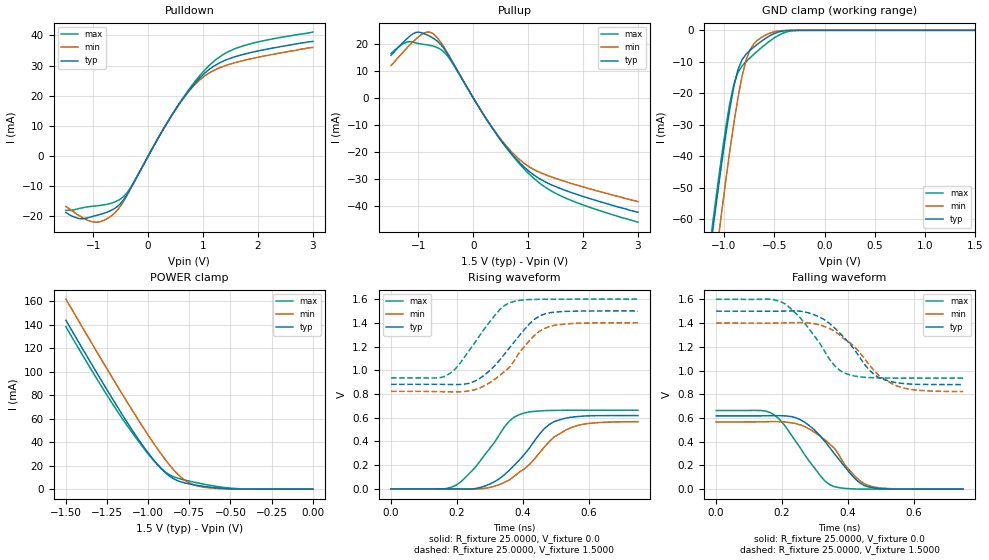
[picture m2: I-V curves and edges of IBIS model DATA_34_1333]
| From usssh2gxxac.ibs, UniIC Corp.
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|   Model DATA_34_1333
[Model]  DATA_34_1333
Model_type I/O
Polarity   Non-Inverting
Enable   Active-High
Vinl =   0.60000000V
Vinh =   0.90000000V
Vmeas =   0.750000000V
Rref =   25.00000000
Vref =   0.75000000V
C_comp   1.6160pF   1.5990pF   1.6430pF
[Temperature Range]   25.0000   95.0000   0.0
[Voltage Range]   1.5000V   1.4000V   1.6000V
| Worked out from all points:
|   slope of the pulldown table from 0 to 0.225 V, typ, clamps not added: 30.8 ohm
|   slope of the pullup table from 0 to 0.225 V, typ, clamps not added: 30.4 ohm
|   GND clamp passes 1 mA (typ) near -0.50 V on its own axis
|   POWER clamp passes 1 mA (typ) near -0.58 V on its own axis
|   rising waveform, R_fixture 25.0000, V_fixture 0.0: 20-80 % time 115ps typ, 128ps min, 108ps max; typ from 0 V to 0.618 V
|   rising waveform, R_fixture 25.0000, V_fixture 1.5000: 20-80 % time 113ps typ, 111ps min, 104ps max; typ from 0.881 V to 1.5 V
|   falling waveform, R_fixture 25.0000, V_fixture 0.0: 20-80 % time 110ps typ, 107ps min, 101ps max; typ from 0.618 V to 0 V
|   falling waveform, R_fixture 25.0000, V_fixture 1.5000: 20-80 % time 112ps typ, 125ps min, 105ps max; typ from 1.5 V to 0.882 V
[Pulldown]
|Voltage   I(typ)   I(min)   I(max)
-1.5V     -18.7mA    -16.7mA    -18mA
-1.25V    -20.76mA   -19.8mA    -17.33mA
-1V       -19.96mA   -21.85mA   -16.61mA
-800mV    -18.94mA   -21.24mA   -16.16mA
-600mV    -17.23mA   -18.69mA   -15.15mA
-350mV    -11.62mA   -11.84mA   -11.29mA
200mV     6.523mA    6.58mA     6.518mA
550mV     16.83mA    16.81mA    16.97mA
850mV     24.09mA    23.66mA    24.66mA
1.15V     29.22mA    27.95mA    30.67mA
1.7V      33.54mA    31.52mA    36.35mA
3V        38mA       36mA       41.1mA
[Pullup]
|Voltage   I(typ)   I(min)   I(max)
-1.5V     15.8mA     12mA       16.5mA
-1.25V    21.14mA    17.6mA     20.39mA
-1.05V    24.23mA    21.76mA    20.4mA
-900mV    23.84mA    24.02mA    19.83mA
-750mV    22.38mA    24mA       19.29mA
-600mV    19.94mA    20.83mA    18.05mA
-450mV    15.66mA    15.92mA    15.03mA
300mV     -9.744mA   -9.622mA   -9.709mA
850mV     -24.07mA   -22.95mA   -24.6mA
1.2V      -29.82mA   -27.44mA   -31.4mA
1.55V     -33.24mA   -30.13mA   -35.83mA
3V        -42.3mA    -38.4mA    -46mA
[GND_clamp]
|Voltage   I(typ)   I(min)   I(max)
-1.5V     -169mA     -189.1mA   -163.8mA
-1.14V    -70.71mA   -88.3mA    -68.32mA
-1.1V     -60.74mA   -77.66mA   -58.33mA
-1.06V    -51.03mA   -67.22mA   -48.61mA
-1.02V    -41.65mA   -57.06mA   -39.27mA
-940mV    -24.55mA   -37.9mA    -22.88mA
-860mV    -12.39mA   -21.26mA   -13.32mA
-780mV    -7.577mA   -9.433mA   -9.942mA
-740mV    -6.329mA   -6.125mA   -8.71mA
-620mV    -3.273mA   -2.113mA   -5.305mA
-300mV    -11.81uA   -4.878uA   -91.71uA
1.5V      4.577nA    23.6nA     33.33nA
[POWER_clamp]
|Voltage   I(typ)   I(min)   I(max)
-1.5V     143.7mA    161.7mA    138.1mA
-1.22V    77.56mA    95.29mA    73.32mA
-1.12V    55.19mA    72.34mA    52.54mA
-1.02V    34.59mA    50.23mA    33.56mA
-960mV    23.77mA    37.63mA    23.28mA
-900mV    14.66mA    25.9mA     15mA
-840mV    8.415mA    15.63mA    10.28mA
-780mV    5.408mA    7.848mA    7.861mA
-700mV    3.206mA    2.693mA    5.332mA
-600mV    1.29mA     794.5uA    2.681mA
-420mV    69.47uA    44.47uA    238.7uA
0V        4.577nA    6.249nA    39.08nA
[Ramp]
| variable   typ   min   max
dV/dt_r  0.3707/0.1151n   0.3398/0.1312n   0.3978/0.1081n
dV/dt_f  0.3712/0.1121n   0.3468/0.1264n   0.3986/0.1049n
R_load = 25.0000
[Rising Waveform]
R_fixture= 25.0000
V_fixture= 0.0
V_fixture_min= 0.0
V_fixture_max= 0.0
|time   V(typ)   V(min)   V(max)
0s        0V         0V         0V
195ps     -137.5uV   -505.3uV   27.18mV
255ps     2.544mV    -2.401mV   178.8mV
315ps     61.22mV    22.19mV    395mV
360ps     158.9mV    75.74mV    573.3mV
405ps     290.2mV    168.8mV    639.6mV
465ps     505.8mV    350.4mV    659.2mV
495ps     566.8mV    436.6mV    661.4mV
590ps     614.4mV    547.4mV    662.9mV
750ps     617.9mV    566.4mV    663mV
[Rising Waveform]
R_fixture= 25.0000
V_fixture= 1.5000
V_fixture_min= 1.4000
V_fixture_max= 1.6000
|time   V(typ)   V(min)   V(max)
0s        881.4mV    822mV      935.7mV
150ps     881mV      819.6mV    937.7mV
180ps     879.7mV    817.7mV    975.2mV
240ps     891.6mV    826.5mV    1.176V
270ps     932.4mV    850.9mV    1.296V
330ps     1.085V     955.3mV    1.51V
360ps     1.189V     1.025V     1.569V
435ps     1.428V     1.292V     1.597V
480ps     1.483V     1.368V     1.599V
750ps     1.5V       1.4V       1.6V
[Falling Waveform]
R_fixture= 25.0000
V_fixture= 0.0
V_fixture_min= 0.0
V_fixture_max= 0.0
|time   V(typ)   V(min)   V(max)
0s        617.9mV    566.4mV    663mV
135ps     617.9mV    567.7mV    662.9mV
180ps     619mV      569.3mV    618.1mV
210ps     617.7mV    566mV      530.5mV
270ps     561.8mV    525.5mV    285.5mV
330ps     403.3mV    416.2mV    69.54mV
360ps     295.8mV    341.6mV    20.56mV
420ps     92.81mV    113.3mV    2.08mV
465ps     17.27mV    28.24mV    381.4uV
750ps     0V         0V         0V
[Falling Waveform]
R_fixture= 25.0000
V_fixture= 1.5000
V_fixture_min= 1.4000
V_fixture_max= 1.6000
|time   V(typ)   V(min)   V(max)
0s        1.5V       1.4V       1.6V
165ps     1.499V     1.399V     1.601V
210ps     1.501V     1.401V     1.56V
315ps     1.449V     1.384V     1.228V
360ps     1.358V     1.331V     1.04V
405ps     1.228V     1.236V     963.5mV
465ps     1.004V     1.047V     940.4mV
495ps     938.3mV    955.6mV    937.6mV
575ps     889mV      849mV      935.9mV
750ps     881.5mV    822.1mV    935.7mV
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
